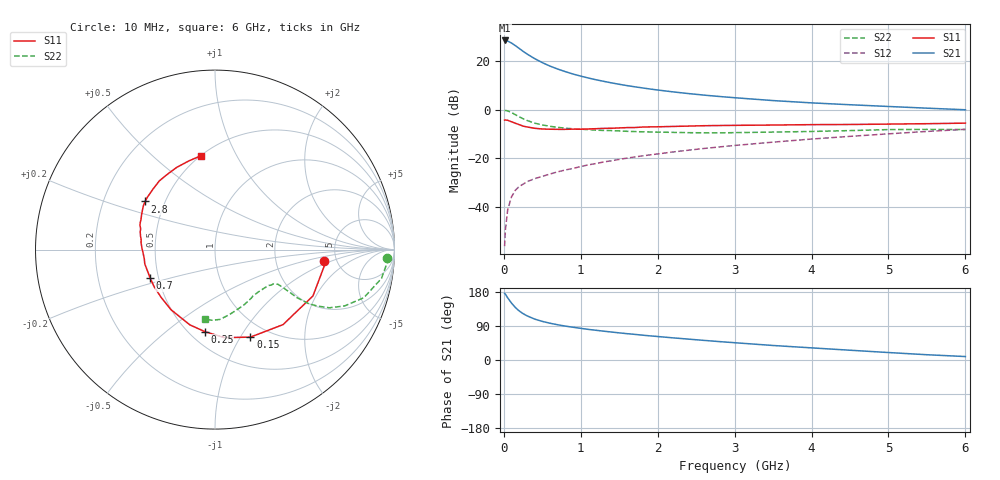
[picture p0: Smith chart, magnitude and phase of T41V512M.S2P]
! Infineon Technologies  Discrete & RF Semiconductors
! BFR182T
! Si NPN RF Bipolar Junction Transistor in SC75
! VCE = 1.5 V  IC = 12 mA
! Common Emitter S-Parameters:  October  1999
# GHz  S  MA  R  50
!  f  S11  S21  S12  S22
! GHz  MAG  ANG  MAG  ANG  MAG  ANG  MAG  ANG
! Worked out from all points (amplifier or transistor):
!   36 points, 10 MHz to 6 GHz, reference 50 ohm
!   highest |S21| = 28.3 dB at 10 MHz (marker M1)
!   |S21| within 3 dB of that: start of sweep to 187.9 MHz
!   unconditionally stable (mu >= 1): 764.4 MHz to 3.882 GHz
!   at 250 MHz: K = 0.54, MSG = 27.2 dB, |S12| = -30.5 dB
!   at 1.4 GHz: K = 1.13, MAG = 13.8 dB, |S12| = -20.9 dB
!   at 6 GHz: K = 0.86, MSG = 4.0 dB, |S12| = -8.1 dB
!   S11 on the Smith chart (normalised r, x): 10 MHz: 3.95, -0.83; 150 MHz: 0.82, -1.11; 250 MHz: 0.59, -0.69; 700 MHz: 0.45, -0.17; 2.8 GHz: 0.39, +0.27; 6 GHz: 0.50, +0.73
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0.01  0.611 -6.2  26.08 175.9  0.0016 84.3  0.9613 -2.7
0.02  0.6147 -8.9  25.94 173.7  0.0034 94.3  0.9638 -3.9
0.05  0.6038 -25.3  25.35 164.0  0.0089 86.5  0.9416 -9.8
0.1  0.5642 -47.8  23.05 150.1  0.0164 72.2  0.8717 -17.9
0.15  0.526 -68.0  20.41 138.4  0.0224 65.1  0.7873 -23.5
0.2  0.4931 -84.0  17.88 129.4  0.0267 62.0  0.7144 -27.0
0.25  0.4601 -97.2  15.65 122.4  0.0297 58.7  0.6497 -28.9
0.3  0.4422 -108.4  13.82 116.7  0.0334 58.2  0.6017 -30.0
0.4  0.415 -126.2  11.09 108.0  0.0386 57.9  0.5287 -30.4
0.5  0.401 -138.7  9.176 101.9  0.043 59.0  0.4861 -29.8
0.6  0.3973 -148.6  7.785 97.0  0.048 59.8  0.4557 -29.5
0.7  0.3946 -156.4  6.777 93.0  0.0533 61.5  0.4333 -29.0
0.9  0.3992 -168.4  5.35 86.4  0.0626 64.3  0.4046 -28.9
1.1  0.4021 -178.0  4.435 80.7  0.0742 64.8  0.3885 -29.7
1.3  0.4134 174.9  3.791 76.0  0.085 66.2  0.3747 -31.0
1.6  0.4286 166.5  3.107 69.5  0.1015 67.1  0.3598 -33.7
2.2  0.4526 154.7  2.308 58.4  0.1359 67.3  0.3424 -41.5
2.8  0.4727 145.4  1.859 48.6  0.172 66.1  0.334 -50.5
3.5  0.4833 135.2  1.532 38.3  0.216 63.8  0.347 -61.6
4.5  0.4964 122.4  1.259 25.8  0.2837 58.7  0.3723 -78.2
5.5  0.5152 106.4  1.071 13.9  0.3574 52.4  0.394 -92.3
6  0.5289 98.6  0.994 9.1  0.3952 48.5  0.3917 -98.4
